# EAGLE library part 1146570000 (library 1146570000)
PCB plug-in connector, male header, open side, THT solder connection, 5.08 mm, Number of poles: 12, 180, Solder pin length: 3.2 mm, tinned, orange, Box Source: Datasheet
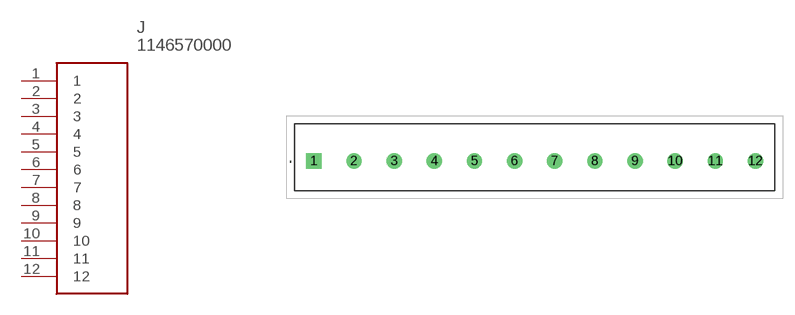
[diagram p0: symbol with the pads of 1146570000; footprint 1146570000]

Designator prefix J

## 1146570000 (Description: PCB plug-in connector, male header, open side, THT solder connection, 5.08 mm, Number of poles: 12, 180, Solder pin length: 3.2 mm, tinned, orange, Box; Height: 12mm; Manufacturer_Name: Weidmuller; Manufacturer_Part_Number: 1146570000; Mouser_Part_Number: 470-1146570000; Mouser_Price-Stock: https://www.mouser.co.uk/ProductDetail/Weidmuller/1146570000?qs=WJDKaGZ8K%252B7cP7z9TJi1CA%3D%3D)  [1146570000]
1  1
2  2
3  3
4  4
5  5
6  6
7  7
8  8
9  9
10  10
11  11
12  12

## Footprint 1146570000 (pad centres in mm)
1146570000
drill 1.3 pad 1.95 square: 1 0,0
drill 1.3 pad 1.95: 2 5.08,0; 3 10.16,0; 4 15.24,0; 5 20.32,0; 6 25.4,0; 7 30.48,0; 8 35.56,0; 9 40.64,0; 10 45.72,0; 11 50.8,0; 12 55.88,0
